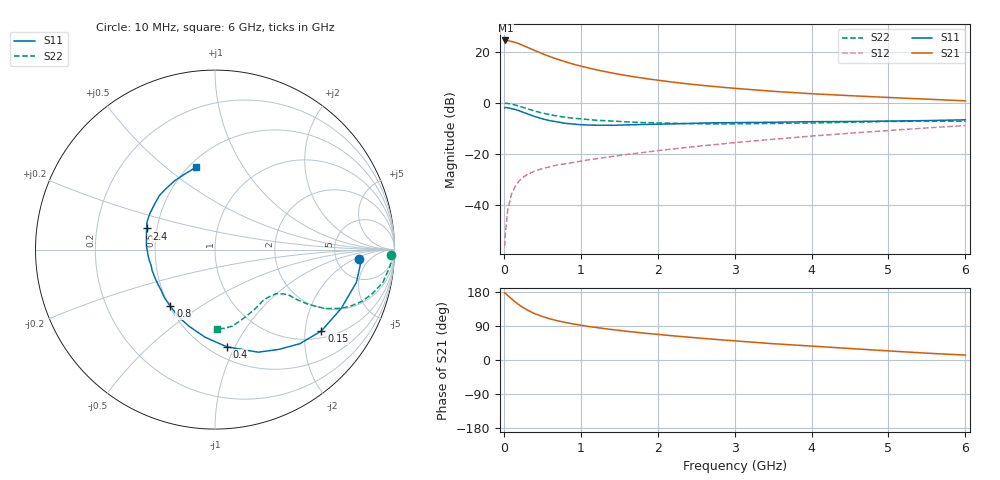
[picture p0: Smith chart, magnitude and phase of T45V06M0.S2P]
! Infineon Technologies  Discrete & RF Semiconductors
! BFR182T
! Si NPN RF Bipolar Junction Transistor in SC75
! VCE = 5 V  IC = 6 mA
! Common Emitter S-Parameters:  October  1999
# GHz  S  MA  R  50
!  f  S11  S21  S12  S22
! GHz  MAG  ANG  MAG  ANG  MAG  ANG  MAG  ANG
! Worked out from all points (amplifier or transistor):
!   36 points, 10 MHz to 6 GHz, reference 50 ohm
!   highest |S21| = 24.4 dB at 20 MHz (marker M1)
!   |S21| within 3 dB of that: start of sweep to 330.5 MHz
!   unconditionally stable (mu >= 1): 1.34 GHz to 3.986 GHz
!   at 250 MHz: K = 0.31, MSG = 25.8 dB, |S12| = -29.0 dB
!   at 1.4 GHz: K = 1.02, MAG = 15.5 dB, |S12| = -20.9 dB
!   at 6 GHz: K = 0.85, MSG = 4.8 dB, |S12| = -8.8 dB
!   lowest NFmin = 1.25 dB at 450 MHz
!   S11 on the Smith chart (normalised r, x): 10 MHz: 8.56, -2.46; 150 MHz: 1.19, -2.44; 400 MHz: 0.60, -0.93; 800 MHz: 0.51, -0.38; 2.4 GHz: 0.44, +0.12; 6 GHz: 0.54, +0.64
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0.01  0.8054 -3.6  16.66 177.1  0.0016 77.1  0.9813 -1.9
0.02  0.8175 -4.0  16.68 176.2  0.0028 95.3  0.99 -2.3
0.05  0.8088 -13.0  16.51 170.4  0.0081 86.6  0.9783 -5.7
0.1  0.7761 -24.9  15.95 161.6  0.0168 79.9  0.9535 -11.0
0.15  0.7462 -37.4  15.21 152.8  0.0237 71.6  0.9118 -15.5
0.2  0.7058 -48.0  14.34 145.2  0.0302 68.5  0.8684 -19.4
0.25  0.6596 -57.5  13.3 138.5  0.0353 64.0  0.82 -22.5
0.3  0.6204 -67.1  12.35 132.5  0.0398 61.4  0.7772 -24.9
0.4  0.546 -83.0  10.65 122.4  0.047 57.1  0.698 -28.1
0.5  0.4913 -96.5  9.207 114.9  0.0525 55.7  0.6382 -29.5
0.6  0.4514 -108.5  8.044 108.5  0.057 54.1  0.5915 -30.6
0.7  0.4259 -118.8  7.133 103.5  0.0618 54.4  0.5553 -31.1
0.8  0.4011 -128.2  6.395 99.0  0.0651 54.4  0.5282 -31.4
0.9  0.3888 -136.6  5.764 95.2  0.0689 54.9  0.5049 -31.6
1.1  0.3711 -150.5  4.834 88.5  0.0776 56.1  0.475 -32.1
1.6  0.3741 -175.0  3.427 75.7  0.0991 59.3  0.429 -34.8
2.2  0.3916 167.3  2.556 63.8  0.127 61.7  0.4026 -40.4
2.4  0.3987 162.8  2.358 60.3  0.1368 62.1  0.396 -42.7
3.5  0.4214 142.9  1.693 43.0  0.1955 61.7  0.3995 -56.5
4.5  0.4358 128.7  1.393 30.3  0.2571 58.8  0.4213 -70.6
5.5  0.4541 111.4  1.189 18.0  0.3262 54.1  0.4419 -83.2
6  0.4706 103.1  1.103 12.9  0.3635 50.8  0.4413 -88.4
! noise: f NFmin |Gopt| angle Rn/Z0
0.45  1.25  0.25  39  0.3
0.9  1.4  0.25  78  0.23
1.8  1.95  0.21  151  0.2
